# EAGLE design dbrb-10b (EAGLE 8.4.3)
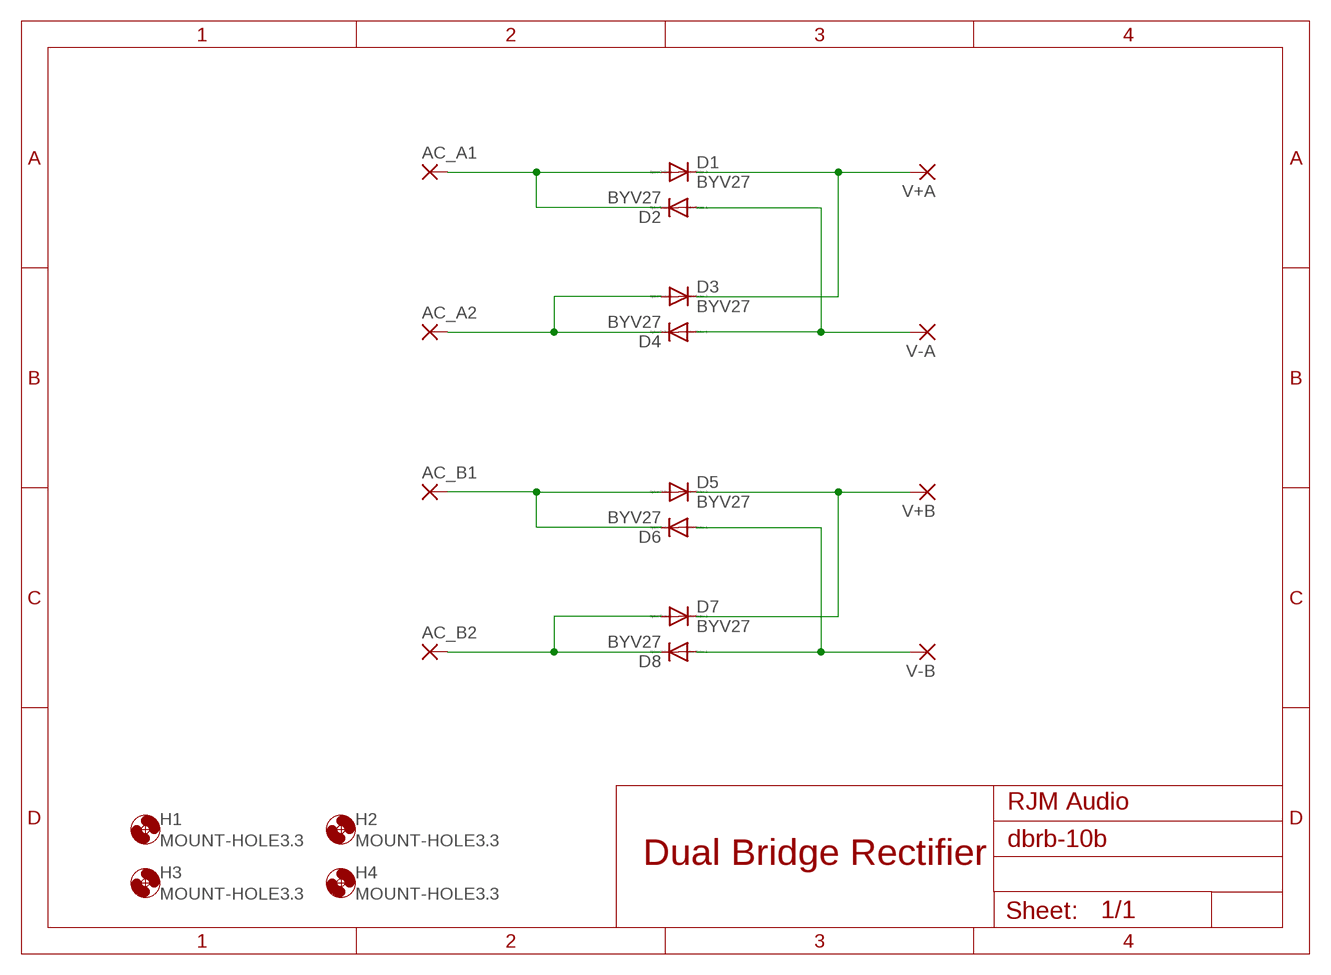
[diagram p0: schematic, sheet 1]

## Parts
AC_A1  3,17/1,3  [3,17/1,3]
AC_A2  3,17/1,3  [3,17/1,3]
AC_B1  3,17/1,3  [3,17/1,3]
AC_B2  3,17/1,3  [3,17/1,3]
D1  BYV27  [SOD57-10]
D2  BYV27  [SOD57-10]
D3  BYV27  [SOD57-10]
D4  BYV27  [SOD57-10]
D5  BYV27  [SOD57-10]
D6  BYV27  [SOD57-10]
D7  BYV27  [SOD57-10]
D8  BYV27  [SOD57-10]
H1  MOUNT-HOLE3.3  [3,3]
H2  MOUNT-HOLE3.3  [3,3]
H3  MOUNT-HOLE3.3  [3,3]
H4  MOUNT-HOLE3.3  [3,3]
V+A  3,17/1,3  [3,17/1,3]
V+B  3,17/1,3  [3,17/1,3]
V-A  3,17/1,3  [3,17/1,3]
V-B  3,17/1,3  [3,17/1,3]

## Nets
A1: AC_A1.1(P) D1.A D2.C
A2: AC_A2.1(P) D3.A D4.C
B1: AC_B1.1(P) D5.A D6.C
B2: AC_B2.1(P) D7.A D8.C
V+A: D1.C D3.C V+A.1(P)
V+B: D5.C D7.C V+B.1(P)
V-A: D2.A D4.A V-A.1(P)
V-B: D6.A D8.A V-B.1(P)

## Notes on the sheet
- RJM Audio
- Dual Bridge Rectifier

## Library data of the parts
AC_A1 AC_A2 AC_B1 AC_B2 V+A V+B V-A V-B = wirepad:3,17/1,3: THROUGH-HOLE PAD
D1-D8 = diode:BYV27: DIODE
H1-H4 = holes:MOUNT-HOLE: MOUNTING HOLE with drill center marker

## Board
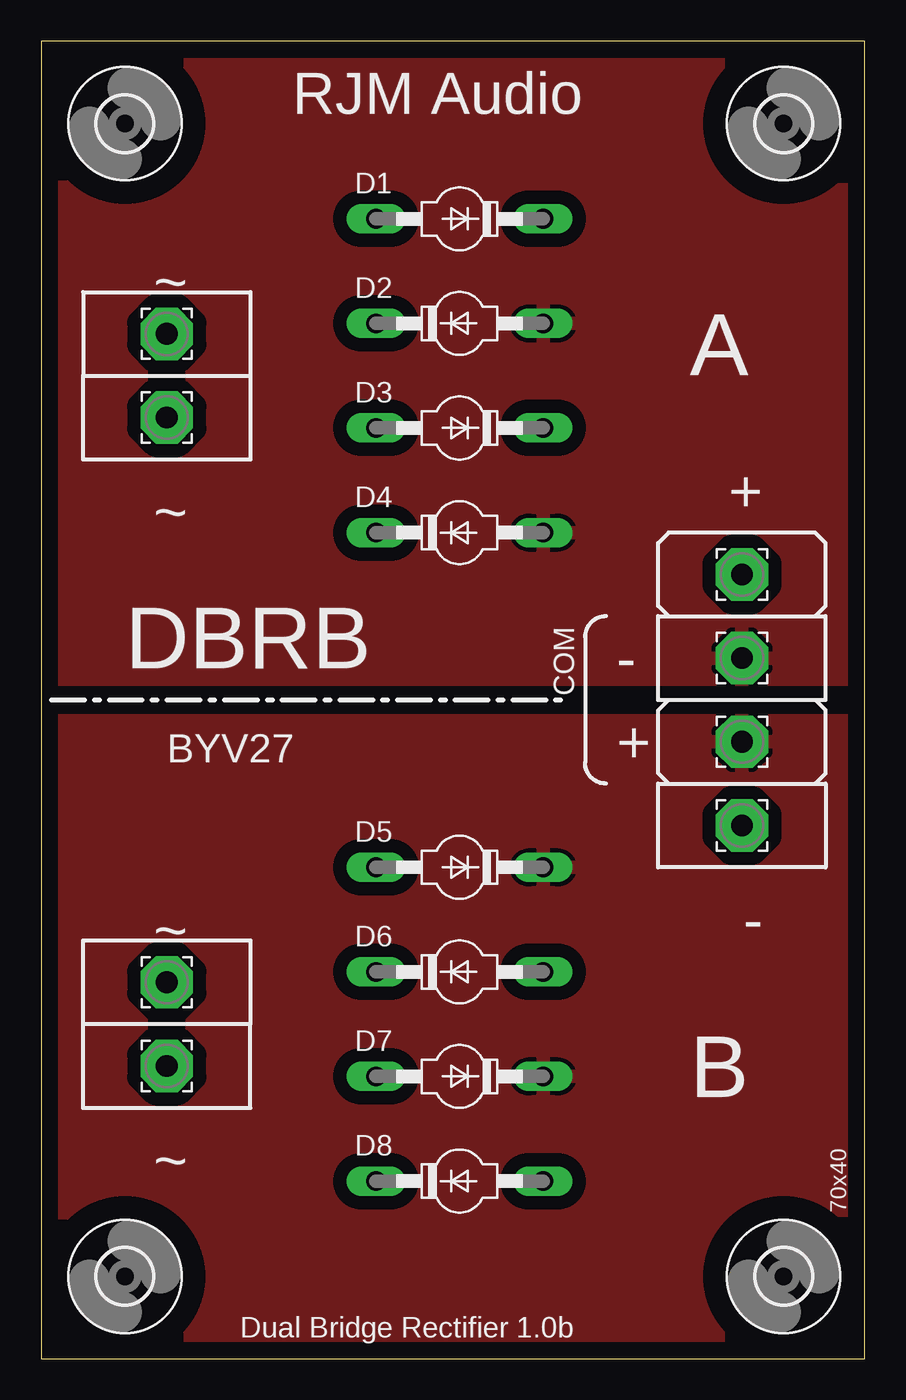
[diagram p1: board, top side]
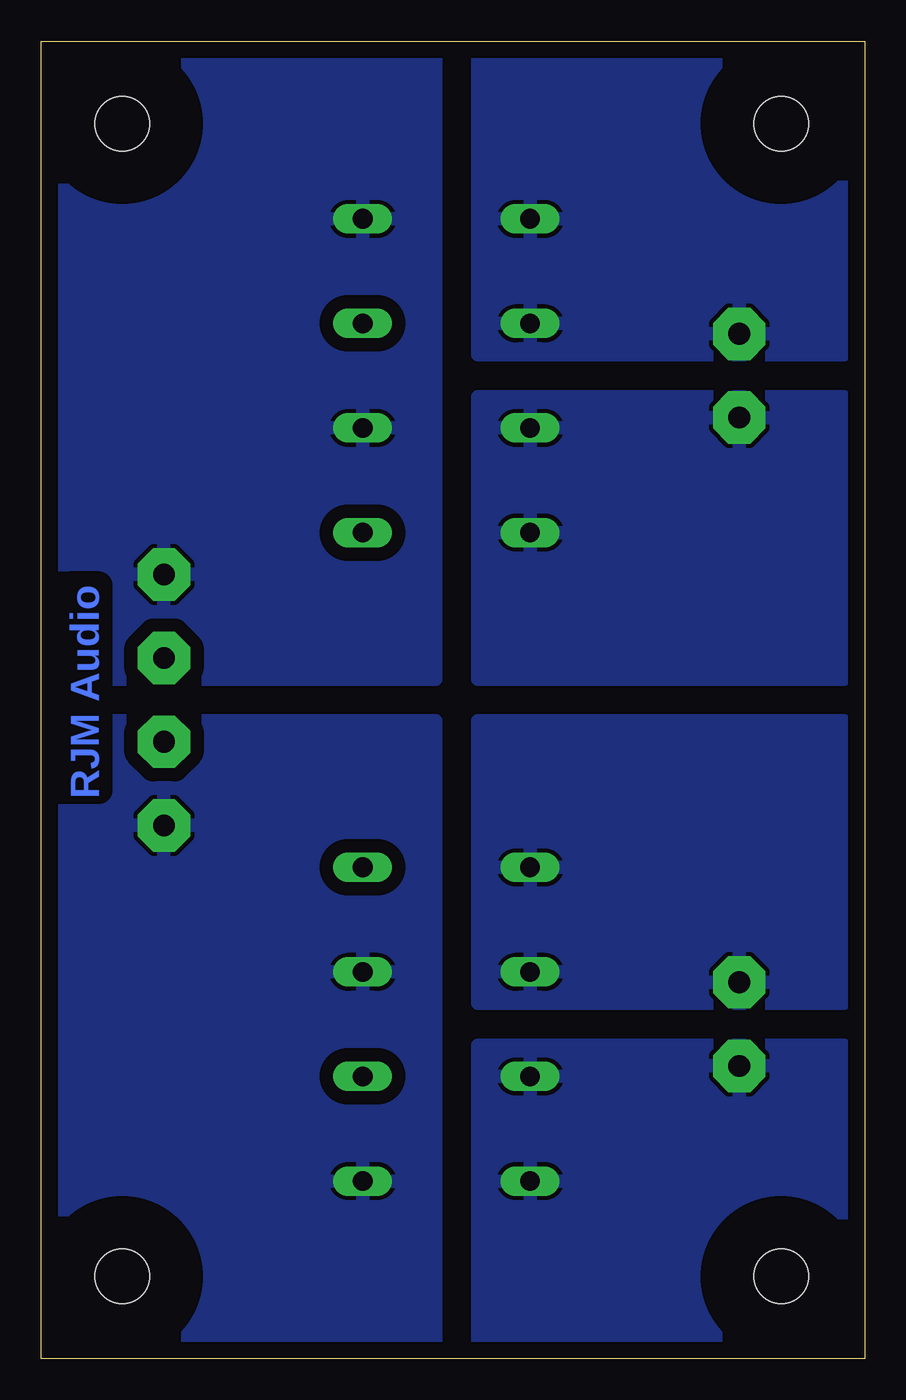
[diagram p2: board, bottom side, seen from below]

Size 50 x 80 mm. Coordinates in mm from the lower left corner, seen from the top.
Outline: 0,0 50,0 50,80 0,80 0,0
Copper layers (1*16): Top 0.035mm / dielectric 1.5mm / Bottom 0.035mm
Design rules "default": minimum track width 10mil, minimum drill 24mil, track to track 8mil, track to pad 8mil, pad to pad 8mil, via to via 8mil, smd to smd 8mil, copper to edge 40mil, drill to drill 8mil, minimum pad ring 10mil, minimum via ring 8mil, stop-mask expansion 4mil, vias tented up to drill 0mil, thermal gap 10mil

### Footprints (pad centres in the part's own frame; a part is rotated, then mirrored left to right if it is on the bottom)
3,17/1,3 = drill 1.321 pad 3.175 octagon: 1 0,0
SOD57-10 = drill 1.194 long: A 5.08,0; C -5.08,0
3,3 = hole 3.3: 0,0

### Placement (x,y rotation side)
AC_A1  7.62,62.23 0 top
AC_A2  7.62,57.15 0 top
AC_B1  7.62,22.86 0 top
AC_B2  7.62,17.78 0 top
D1  25.4,69.21 180 top
D2  25.4,62.87 0 top
D3  25.4,56.52 180 top
D4  25.4,50.16 0 top
D5  25.4,29.84 180 top
D6  25.4,23.49 0 top
D7  25.4,17.14 180 top
D8  25.4,10.79 0 top
H1  5.08,75 0 top
H2  45.08,75 0 top
H3  5.08,5 0 top
H4  45.08,5 0 top
V+A  42.55,47.62 0 top
V+B  42.55,37.47 0 top
V-A  42.55,42.55 0 top
V-B  42.55,32.39 0 top

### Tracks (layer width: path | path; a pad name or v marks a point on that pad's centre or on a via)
A1
  pour Bottom (isolate 0.813): 1.27,60.96 23.5,60.96 23.5,79.38 1.27,79.38
A2
  pour Bottom (isolate 0.813): 1.27,58.42 23.5,58.42 23.5,41.27 1.27,41.27
B1
  pour Bottom (isolate 0.813): 1.27,38.73 23.5,38.73 23.5,21.59 1.27,21.59
B2
  pour Bottom (isolate 0.813): 1.27,19.05 23.5,19.05 23.5,0.64 1.27,0.64
V+A
  pour Bottom (isolate 0.813, rank 3): 26.04,41.27 26.04,79.38 49.53,79.38 49.53,41.27
V+B
  pour Top (isolate 0.813): 0,38.73 0,-0.64 50.16,-0.64 50.16,38.73
V-A
  pour Top (isolate 0.813): 0,80.01 50.16,80.01 50.16,41.27 0,41.27
V-B
  pour Bottom (isolate 0.813, rank 3): 26.04,38.73 49.53,38.73 49.53,0.64 26.04,0.64

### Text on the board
Bottom: RJM Audio
tPlace: RJM Audio | ~ | A | + | ~ | COM | DBRB | - | BYV27 | + | - | ~ | B | ~ | 70x40 | Dual Bridge Rectifier 1.0b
